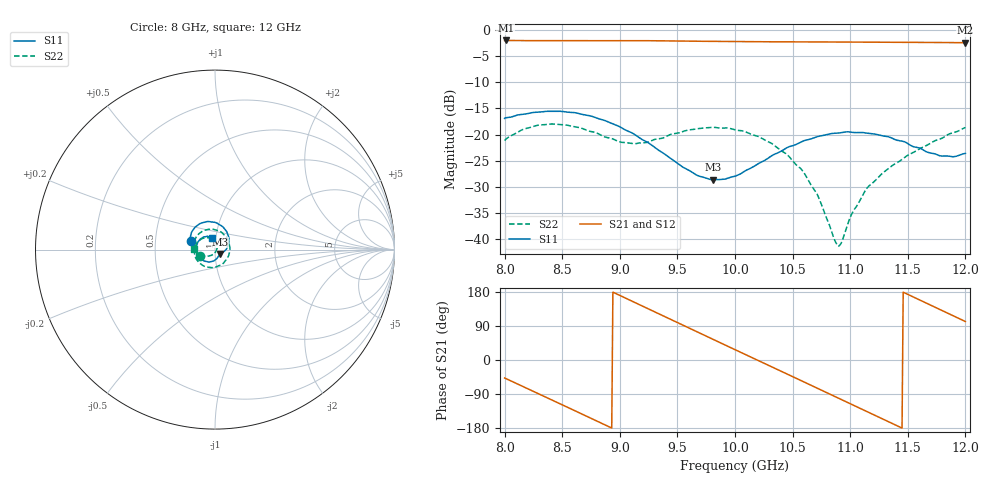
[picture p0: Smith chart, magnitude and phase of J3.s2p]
!Keysight Technologies,N5234A,MY52241180,A.10.60.03
!Date: Tuesday, May 30, 2023 15:19:23
!Correction: S11(Full 2 Port(1,2))
!S21(Full 2 Port(1,2))
!S12(Full 2 Port(1,2))
!S22(Full 2 Port(1,2))
!S2P File: Measurements: S11, S21, S12, S22:
# Hz S  dB  R 50
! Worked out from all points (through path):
!   401 points, 8 GHz to 12 GHz, reference 50 ohm
!   highest |S21| = -2.01 dB at 8.01 GHz (marker M1); lowest = -2.4 dB at 12 GHz (marker M2)
!   group delay of S21, straight-line fit = 397 ps
!   lowest |S11| = -28.6 dB at 9.81 GHz (marker M3), VSWR 1.08, Z = 52.8 - j2.57 ohm
!   |S11| at or under -10 dB: start of sweep to end of sweep
!   |S22| runs from -41.3 to -18.0 dB; largest |S21 - S12| = 0.0015
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8e9  -16.89 159.6  -2.07 -47.5  -2.07 -47.5  -21.13 -157.7
8.01e9  -16.77 159.2  -2.01 -48.8  -2.02 -48.8  -20.87 -159.0
8.17e9  -16.09 149.3  -2.03 -71.5  -2.05 -71.5  -18.92 179.0
8.33e9  -15.63 135.7  -2.05 -94.2  -2.06 -94.2  -18.12 155.4
8.49e9  -15.55 118.9  -2.05 -116.8  -2.06 -116.8  -18.09 130.1
8.67e9  -16.11 98.6  -2.04 -142.4  -2.06 -142.4  -18.78 97.3
8.84e9  -17.10 77.8  -2.04 -166.7  -2.04 -166.7  -20.14 61.9
9e9  -18.50 56.6  -2.03 170.4  -2.04 170.4  -21.38 22.0
9.16e9  -20.44 35.5  -2.04 147.4  -2.05 147.4  -21.64 -23.1
9.34e9  -23.02 11.7  -2.07 121.5  -2.08 121.5  -20.79 -70.7
9.57e9  -26.47 -17.3  -2.12 88.6  -2.13 88.5  -19.24 -119.5
9.81e9  -28.61 -40.9  -2.19 54.3  -2.20 54.3  -18.59 -160.4
1e10  -27.94 -59.3  -2.23 27.3  -2.23 27.3  -19.07 170.3
1.016e10  -26.11 -76.0  -2.25 4.6  -2.26 4.6  -20.06 147.7
1.032e10  -24.00 -95.5  -2.26 -18.2  -2.28 -18.2  -21.69 125.6
1.067e10  -20.73 -142.8  -2.29 -68.1  -2.30 -68.1  -29.93 73.9
1.09e10  -19.69 -174.6  -2.31 -100.9  -2.32 -101.0  -41.30 -27.3
1.113e10  -19.68 156.3  -2.33 -133.9  -2.33 -133.9  -30.71 -111.8
1.134e10  -20.47 132.4  -2.35 -163.9  -2.36 -163.9  -26.30 -133.0
1.164e10  -23.01 108.6  -2.38 153.1  -2.39 153.1  -22.30 -155.1
1.183e10  -24.08 105.7  -2.40 125.9  -2.41 125.9  -20.22 -168.2
1.2e10  -23.57 104.8  -2.43 101.5  -2.44 101.5  -18.64 178.2
